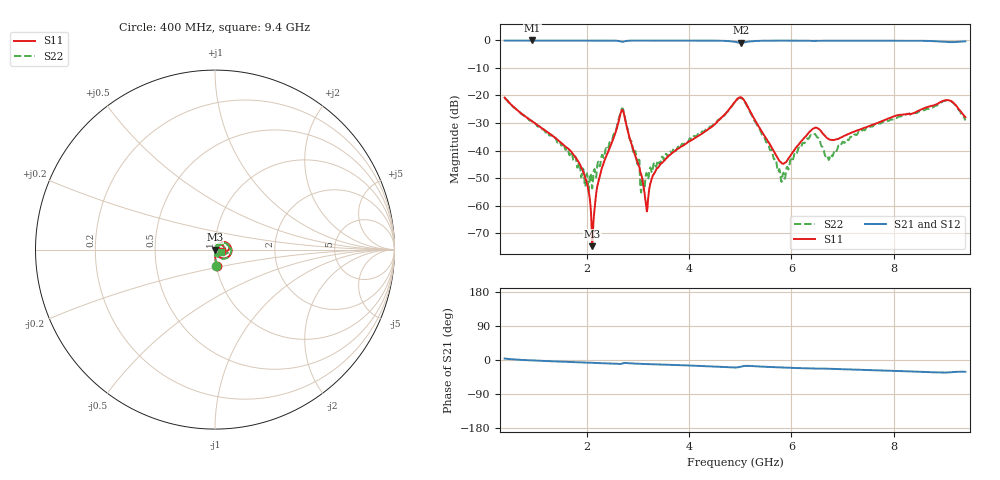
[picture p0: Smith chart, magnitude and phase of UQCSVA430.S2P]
!  Part Number  UQCSVA430  Mounting Orientation: Horizontal
!  Description: Ultra Low ESR Microwave capacitors
!  Application: Coupling, Bypass, Tuning, DC Block
!  Filters, Matching
# GHZ S DB R 50
! Freq  |S11|  S11 Ph  |S21|  S21 Ph  |S12|  S12 Ph  |S22|  S22 Ph
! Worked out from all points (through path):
!   801 points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, 400 MHz to 9.4 GHz, reference 50 ohm
!   highest |S21| = -0.02 dB at 940 MHz (marker M1); lowest = -0.9 dB at 5.013 GHz (marker M2)
!   group delay of S21, straight-line fit = 10.4 ps
!   lowest |S11| = -74.7 dB at 2.11 GHz (marker M3), VSWR 1.00, Z = 50 - j0.0138 ohm
!   |S11| at or under -10 dB: start of sweep to end of sweep
!   |S22| runs from -55.3 to -20.8 dB; largest |S21 - S12| = 0.0022
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0.4  -20.75 -84.7  -0.06 3.9  -0.05 3.9  -20.84 -85.2
0.94  -29.44 -88.9  -0.02 -1.2  -0.02 -1.2  -29.55 -89.5
1.593  -38.67 -89.6  -0.03 -4.6  -0.02 -4.7  -39.81 -82.7
1.908  -46.56 -92.1  -0.03 -6.1  -0.02 -6.1  -48.97 -50.2
2.02  -52.84 -91.7  -0.03 -6.6  -0.03 -6.7  -49.58 -41.1
2.11  -74.74 -48.9  -0.03 -7.0  -0.03 -7.1  -53.74 4.0
2.144  -63.71 62.8  -0.03 -7.2  -0.03 -7.2  -47.12 31.0
2.211  -52.90 79.7  -0.04 -7.5  -0.03 -7.6  -45.36 50.5
2.279  -47.75 81.4  -0.04 -7.9  -0.03 -7.9  -43.91 57.2
2.684  -25.49 14.6  -0.49 -10.0  -0.49 -10.0  -24.96 5.5
2.988  -43.97 -97.0  -0.05 -9.8  -0.05 -9.8  -44.74 -62.7
3.089  -50.34 -61.8  -0.05 -10.3  -0.04 -10.3  -50.85 0.9
3.156  -58.78 -33.0  -0.05 -10.6  -0.04 -10.7  -49.13 36.0
3.404  -46.04 65.3  -0.05 -11.8  -0.04 -11.8  -43.61 50.5
4.9  -22.24 26.6  -0.53 -19.8  -0.53 -19.9  -22.28 23.3
5.013  -20.68 -9.3  -0.87 -17.7  -0.86 -17.7  -20.93 -13.3
5.834  -44.80 -15.5  -0.08 -19.8  -0.08 -19.9  -48.41 -12.4
6.408  -32.30 27.3  -0.17 -22.6  -0.17 -22.7  -34.55 14.5
6.768  -36.12 13.0  -0.10 -23.2  -0.11 -23.3  -41.50 29.2
7.904  -28.32 48.6  -0.09 -28.2  -0.09 -28.3  -29.21 47.7
9.051  -21.68 14.4  -0.57 -32.9  -0.57 -33.0  -21.69 3.7
9.4  -27.90 -10.8  -0.33 -31.1  -0.33 -31.2  -29.06 -20.8
